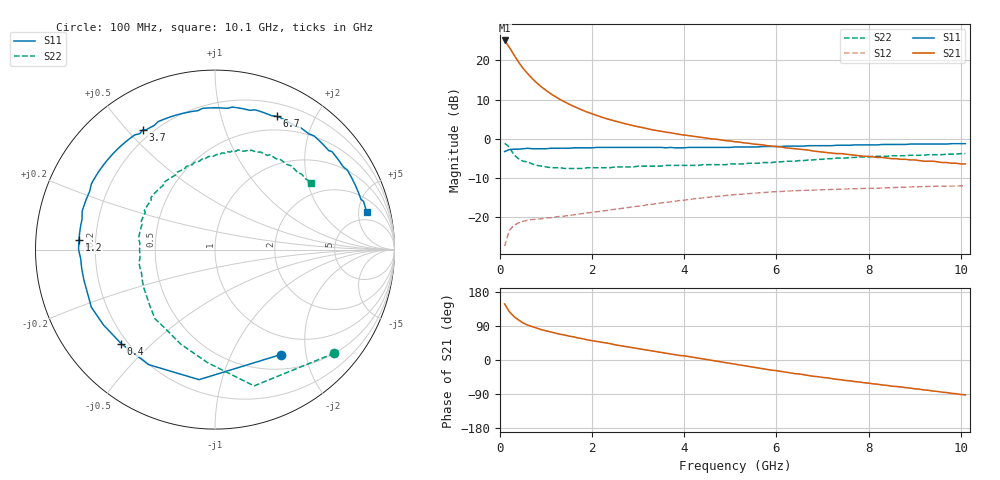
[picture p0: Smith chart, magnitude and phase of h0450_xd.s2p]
!HBFP-0450
!S and NOISE PARAMETERS at Vce=0.5V  Ic=10mA.  LAST UPDATED  09-04-98
# GHZ S MA R  50
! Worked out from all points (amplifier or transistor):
!   101 points, 100 MHz to 10.1 GHz, reference 50 ohm
!   highest |S21| = 25.1 dB at 100 MHz (marker M1)
!   |S21| within 3 dB of that: start of sweep to 267.9 MHz
!   unconditionally stable (mu >= 1): 2.702 GHz to end of sweep
!   at 1.7 GHz: K = 0.78, MSG = 13.5 dB, |S12| = -19.2 dB
!   at 5.1 GHz: K = 1.15, MAG = 4.4 dB, |S12| = -14.2 dB
!   at 10.1 GHz: K = 1.11, MAG = 0.8 dB, |S12| = -12.0 dB
!   lowest NFmin = 1.18 dB at 1.8 GHz
!   S11 on the Smith chart (normalised r, x): 100 MHz: 0.70, -1.57; 400 MHz: 0.17, -0.40; 1.2 GHz: 0.14, +0.03; 3.7 GHz: 0.16, +0.55; 6.7 GHz: 0.33, +1.52; 10.1 GHz: 3.54, +6.14
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0.1  0.69 -58.0  17.97 148.0  0.043 63.0  0.88 -41.0
0.2  0.73 -97.0  14.78 128.0  0.068 47.0  0.79 -74.0
0.3  0.74 -120.0  11.85 115.0  0.079 35.0  0.63 -94.0
0.4  0.74 -135.0  9.58 106.0  0.085 29.0  0.56 -110.0
0.5  0.75 -146.0  7.94 98.0  0.089 25.0  0.52 -122.0
0.6  0.76 -155.0  6.8 92.0  0.092 22.0  0.51 -131.0
0.7  0.75 -162.0  5.87 88.0  0.094 20.0  0.48 -139.0
0.8  0.75 -167.0  5.16 84.0  0.095 19.0  0.46 -146.0
0.9  0.75 -172.0  4.59 80.0  0.096 18.0  0.45 -152.0
1.1  0.76 180.0  3.77 74.0  0.099 17.0  0.43 -162.0
1.2  0.76 176.0  3.46 71.0  0.101 17.0  0.43 -166.0
1.5  0.76 167.0  2.77 63.0  0.106 17.0  0.42 -177.0
1.8  0.77 159.0  2.31 56.0  0.112 16.0  0.42 175.0
2.1  0.78 152.0  1.99 49.0  0.118 16.0  0.43 168.0
2.5  0.78 144.0  1.69 40.0  0.127 14.0  0.44 160.0
3.5  0.78 125.0  1.25 20.0  0.153 8.0  0.45 142.0
3.7  0.78 121.0  1.2 16.0  0.158 7.0  0.46 139.0
5.1  0.79 95.0  0.92 -11.0  0.195 -8.0  0.48 114.0
6.7  0.82 65.0  0.72 -41.0  0.222 -29.0  0.54 86.0
6.8  0.82 63.0  0.7 -43.0  0.223 -31.0  0.54 84.0
8.5  0.85 37.0  0.56 -69.0  0.239 -52.0  0.61 60.0
10.1  0.87 14.0  0.48 -92.0  0.252 -73.0  0.65 35.0
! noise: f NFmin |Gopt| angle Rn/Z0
1.8  1.18  0.53  -179  0.04
2  1.22  0.56  -173  0.04
2.5  1.36  0.57  -159  0.06
3.5  1.65  0.66  -137  0.16
4  1.85  0.67  -125  0.29
5  2.1  0.71  -103  0.61
5.5  2.24  0.74  -92  0.89
7  2.72  0.78  -63  1.96
8  2.96  0.8  -47  2.76
10  3.54  0.81  -16  4.53
